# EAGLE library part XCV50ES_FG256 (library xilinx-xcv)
xcv50es_fg256 edit this description Auto generated by make-symbol-device-package-bsdl.ulp Rev. 26 Source: xcv50es_fg256.bsd
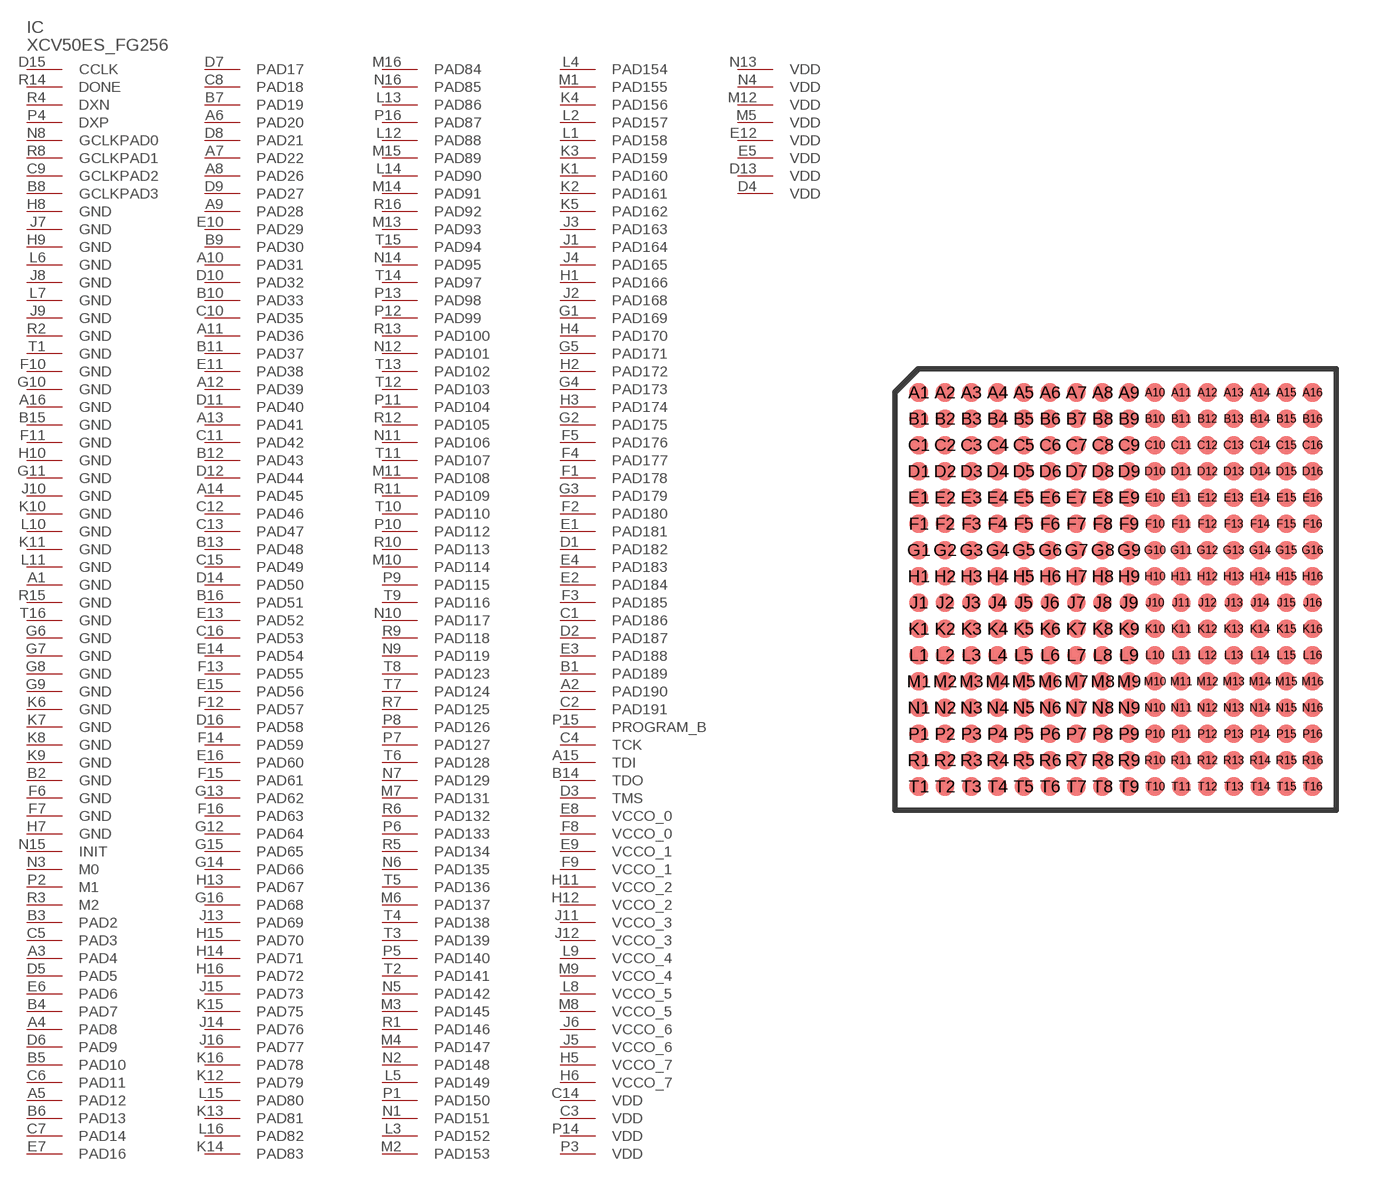
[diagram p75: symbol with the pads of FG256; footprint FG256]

Designator prefix IC

## XCV50ES_FG256 (OC_FARNELL: unknown; OC_NEWARK: unknown)  [FG256]
A1  GND  pwr
A2  PAD190
A3  PAD4
A4  PAD8
A5  PAD12
A6  PAD20
A7  PAD22
A8  PAD26
A9  PAD28
A10  PAD31
A11  PAD36
A12  PAD39
A13  PAD41
A14  PAD45
A15  TDI  in
A16  GND  pwr
B1  PAD189
B2  GND  pwr
B3  PAD2
B4  PAD7
B5  PAD10
B6  PAD13
B7  PAD19
B8  GCLKPAD3  in
B9  PAD30
B10  PAD33
B11  PAD37
B12  PAD43
B13  PAD48
B14  TDO  out
B15  GND  pwr
B16  PAD51
C1  PAD186
C2  PAD191
C3  VDD  pwr
C4  TCK  in
C5  PAD3
C6  PAD11
C7  PAD14
C8  PAD18
C9  GCLKPAD2  in
C10  PAD35
C11  PAD42
C12  PAD46
C13  PAD47
C14  VDD  pwr
C15  PAD49
C16  PAD53
D1  PAD182
D2  PAD187
D3  TMS  in
D4  VDD  pwr
D5  PAD5
D6  PAD9
D7  PAD17
D8  PAD21
D9  PAD27
D10  PAD32
D11  PAD40
D12  PAD44
D13  VDD  pwr
D14  PAD50
D15  CCLK
D16  PAD58
E1  PAD181
E2  PAD184
E3  PAD188
E4  PAD183
E5  VDD  pwr
E6  PAD6
E7  PAD16
E8  VCCO_0  pwr
E9  VCCO_1  pwr
E10  PAD29
E11  PAD38
E12  VDD  pwr
E13  PAD52
E14  PAD54
E15  PAD56
E16  PAD60
F1  PAD178
F2  PAD180
F3  PAD185
F4  PAD177
F5  PAD176
F6  GND  pwr
F7  GND  pwr
F8  VCCO_0  pwr
F9  VCCO_1  pwr
F10  GND  pwr
F11  GND  pwr
F12  PAD57
F13  PAD55
F14  PAD59
F15  PAD61
F16  PAD63
G1  PAD169
G2  PAD175
G3  PAD179
G4  PAD173
G5  PAD171
G6  GND  pwr
G7  GND  pwr
G8  GND  pwr
G9  GND  pwr
G10  GND  pwr
G11  GND  pwr
G12  PAD64
G13  PAD62
G14  PAD66
G15  PAD65
G16  PAD68
H1  PAD166
H2  PAD172
H3  PAD174
H4  PAD170
H5  VCCO_7  pwr
H6  VCCO_7  pwr
H7  GND  pwr
H8  GND  pwr
H9  GND  pwr
H10  GND  pwr
H11  VCCO_2  pwr
H12  VCCO_2  pwr
H13  PAD67
H14  PAD71
H15  PAD70
H16  PAD72
J1  PAD164
J2  PAD168
J3  PAD163
J4  PAD165
J5  VCCO_6  pwr
J6  VCCO_6  pwr
J7  GND  pwr
J8  GND  pwr
J9  GND  pwr
J10  GND  pwr
J11  VCCO_3  pwr
J12  VCCO_3  pwr
J13  PAD69
J14  PAD76
J15  PAD73
J16  PAD77
K1  PAD160
K2  PAD161
K3  PAD159
K4  PAD156
K5  PAD162
K6  GND  pwr
K7  GND  pwr
K8  GND  pwr
K9  GND  pwr
K10  GND  pwr
K11  GND  pwr
K12  PAD79
K13  PAD81
K14  PAD83
K15  PAD75
K16  PAD78
L1  PAD158
L2  PAD157
L3  PAD152
L4  PAD154
L5  PAD149
L6  GND  pwr
L7  GND  pwr
L8  VCCO_5  pwr
L9  VCCO_4  pwr
L10  GND  pwr
L11  GND  pwr
L12  PAD88
L13  PAD86
L14  PAD90
L15  PAD80
L16  PAD82
M1  PAD155
M2  PAD153
M3  PAD145
M4  PAD147
M5  VDD  pwr
M6  PAD137
M7  PAD131
M8  VCCO_5  pwr
M9  VCCO_4  pwr
M10  PAD114
M11  PAD108
M12  VDD  pwr
M13  PAD93
M14  PAD91
M15  PAD89
M16  PAD84
N1  PAD151
N2  PAD148
N3  M0  in
N4  VDD  pwr
N5  PAD142
N6  PAD135
N7  PAD129
N8  GCLKPAD0  in
N9  PAD119
N10  PAD117
N11  PAD106
N12  PAD101
N13  VDD  pwr
N14  PAD95
N15  INIT
N16  PAD85
P1  PAD150
P2  M1  in
P3  VDD  pwr
P4  DXP  pas
P5  PAD140
P6  PAD133
P7  PAD127
P8  PAD126
P9  PAD115
P10  PAD112
P11  PAD104
P12  PAD99
P13  PAD98
P14  VDD  pwr
P15  PROGRAM_B  in
P16  PAD87
R1  PAD146
R2  GND  pwr
R3  M2  in
R4  DXN  pas
R5  PAD134
R6  PAD132
R7  PAD125
R8  GCLKPAD1  in
R9  PAD118
R10  PAD113
R11  PAD109
R12  PAD105
R13  PAD100
R14  DONE
R15  GND  pwr
R16  PAD92
T1  GND  pwr
T2  PAD141
T3  PAD139
T4  PAD138
T5  PAD136
T6  PAD128
T7  PAD124
T8  PAD123
T9  PAD116
T10  PAD110
T11  PAD107
T12  PAD103
T13  PAD102
T14  PAD97
T15  PAD94
T16  GND  pwr

## Footprint FG256 (pad centres in mm)
Fine Pitch BGA (FG256) Auto generated by make-symbol-device-package-bsdl.ulp Rev. 26 Source: xcv100_fg256.bsd; fg256.pdf
smd 0.7 x 0.7: A1 -7.5,7.5; A2 -6.5,7.5; A3 -5.5,7.5; A4 -4.5,7.5; A5 -3.5,7.5; A6 -2.5,7.5; A7 -1.5,7.5; A8 -0.5,7.5; A9 0.5,7.5; A10 1.5,7.5; A11 2.5,7.5; A12 3.5,7.5; A13 4.5,7.5; A14 5.5,7.5; A15 6.5,7.5; A16 7.5,7.5; B1 -7.5,6.5; B2 -6.5,6.5; B3 -5.5,6.5; B4 -4.5,6.5; B5 -3.5,6.5; B6 -2.5,6.5; B7 -1.5,6.5; B8 -0.5,6.5; B9 0.5,6.5; B10 1.5,6.5; B11 2.5,6.5; B12 3.5,6.5; B13 4.5,6.5; B14 5.5,6.5; B15 6.5,6.5; B16 7.5,6.5; C1 -7.5,5.5; C2 -6.5,5.5; C3 -5.5,5.5; C4 -4.5,5.5; C5 -3.5,5.5; C6 -2.5,5.5; C7 -1.5,5.5; C8 -0.5,5.5; C9 0.5,5.5; C10 1.5,5.5; C11 2.5,5.5; C12 3.5,5.5; C13 4.5,5.5; C14 5.5,5.5; C15 6.5,5.5; C16 7.5,5.5; D1 -7.5,4.5; D2 -6.5,4.5; D3 -5.5,4.5; D4 -4.5,4.5; D5 -3.5,4.5; D6 -2.5,4.5; D7 -1.5,4.5; D8 -0.5,4.5; D9 0.5,4.5; D10 1.5,4.5; D11 2.5,4.5; D12 3.5,4.5; D13 4.5,4.5; D14 5.5,4.5; D15 6.5,4.5; D16 7.5,4.5; E1 -7.5,3.5; E2 -6.5,3.5; E3 -5.5,3.5; E4 -4.5,3.5; E5 -3.5,3.5; E6 -2.5,3.5; E7 -1.5,3.5; E8 -0.5,3.5; E9 0.5,3.5; E10 1.5,3.5; E11 2.5,3.5; E12 3.5,3.5; E13 4.5,3.5; E14 5.5,3.5; E15 6.5,3.5; E16 7.5,3.5; F1 -7.5,2.5; F2 -6.5,2.5; F3 -5.5,2.5; F4 -4.5,2.5; F5 -3.5,2.5; F6 -2.5,2.5; F7 -1.5,2.5; F8 -0.5,2.5; F9 0.5,2.5; F10 1.5,2.5; F11 2.5,2.5; F12 3.5,2.5; F13 4.5,2.5; F14 5.5,2.5; F15 6.5,2.5; F16 7.5,2.5; G1 -7.5,1.5; G2 -6.5,1.5; G3 -5.5,1.5; G4 -4.5,1.5; G5 -3.5,1.5; G6 -2.5,1.5; G7 -1.5,1.5; G8 -0.5,1.5; G9 0.5,1.5; G10 1.5,1.5; G11 2.5,1.5; G12 3.5,1.5; G13 4.5,1.5; G14 5.5,1.5; G15 6.5,1.5; G16 7.5,1.5; H1 -7.5,0.5; H2 -6.5,0.5; H3 -5.5,0.5; H4 -4.5,0.5; H5 -3.5,0.5; H6 -2.5,0.5; H7 -1.5,0.5; H8 -0.5,0.5; H9 0.5,0.5; H10 1.5,0.5; H11 2.5,0.5; H12 3.5,0.5; H13 4.5,0.5; H14 5.5,0.5; H15 6.5,0.5; H16 7.5,0.5; J1 -7.5,-0.5; J2 -6.5,-0.5; J3 -5.5,-0.5; J4 -4.5,-0.5; J5 -3.5,-0.5; J6 -2.5,-0.5; J7 -1.5,-0.5; J8 -0.5,-0.5; J9 0.5,-0.5; J10 1.5,-0.5; J11 2.5,-0.5; J12 3.5,-0.5; J13 4.5,-0.5; J14 5.5,-0.5; J15 6.5,-0.5; J16 7.5,-0.5; K1 -7.5,-1.5; K2 -6.5,-1.5; K3 -5.5,-1.5; K4 -4.5,-1.5; K5 -3.5,-1.5; K6 -2.5,-1.5; K7 -1.5,-1.5; K8 -0.5,-1.5; K9 0.5,-1.5; K10 1.5,-1.5; K11 2.5,-1.5; K12 3.5,-1.5; K13 4.5,-1.5; K14 5.5,-1.5; K15 6.5,-1.5; K16 7.5,-1.5; L1 -7.5,-2.5; L2 -6.5,-2.5; L3 -5.5,-2.5; L4 -4.5,-2.5; L5 -3.5,-2.5; L6 -2.5,-2.5; L7 -1.5,-2.5; L8 -0.5,-2.5; L9 0.5,-2.5; L10 1.5,-2.5; L11 2.5,-2.5; L12 3.5,-2.5; L13 4.5,-2.5; L14 5.5,-2.5; L15 6.5,-2.5; L16 7.5,-2.5; M1 -7.5,-3.5; M2 -6.5,-3.5; M3 -5.5,-3.5; M4 -4.5,-3.5; M5 -3.5,-3.5; M6 -2.5,-3.5; M7 -1.5,-3.5; M8 -0.5,-3.5; M9 0.5,-3.5; M10 1.5,-3.5; M11 2.5,-3.5; M12 3.5,-3.5; M13 4.5,-3.5; M14 5.5,-3.5; M15 6.5,-3.5; M16 7.5,-3.5; N1 -7.5,-4.5; N2 -6.5,-4.5; N3 -5.5,-4.5; N4 -4.5,-4.5; N5 -3.5,-4.5; N6 -2.5,-4.5; N7 -1.5,-4.5; N8 -0.5,-4.5; N9 0.5,-4.5; N10 1.5,-4.5; N11 2.5,-4.5; N12 3.5,-4.5; N13 4.5,-4.5; N14 5.5,-4.5; N15 6.5,-4.5; N16 7.5,-4.5; P1 -7.5,-5.5; P2 -6.5,-5.5; P3 -5.5,-5.5; P4 -4.5,-5.5; P5 -3.5,-5.5; P6 -2.5,-5.5; P7 -1.5,-5.5; P8 -0.5,-5.5; P9 0.5,-5.5; P10 1.5,-5.5; P11 2.5,-5.5; P12 3.5,-5.5; P13 4.5,-5.5; P14 5.5,-5.5; P15 6.5,-5.5; P16 7.5,-5.5; R1 -7.5,-6.5; R2 -6.5,-6.5; R3 -5.5,-6.5; R4 -4.5,-6.5; R5 -3.5,-6.5; R6 -2.5,-6.5; R7 -1.5,-6.5; R8 -0.5,-6.5; R9 0.5,-6.5; R10 1.5,-6.5; R11 2.5,-6.5; R12 3.5,-6.5; R13 4.5,-6.5; R14 5.5,-6.5; R15 6.5,-6.5; R16 7.5,-6.5; T1 -7.5,-7.5; T2 -6.5,-7.5; T3 -5.5,-7.5; T4 -4.5,-7.5; T5 -3.5,-7.5; T6 -2.5,-7.5; T7 -1.5,-7.5; T8 -0.5,-7.5; T9 0.5,-7.5; T10 1.5,-7.5; T11 2.5,-7.5; T12 3.5,-7.5; T13 4.5,-7.5; T14 5.5,-7.5; T15 6.5,-7.5; T16 7.5,-7.5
